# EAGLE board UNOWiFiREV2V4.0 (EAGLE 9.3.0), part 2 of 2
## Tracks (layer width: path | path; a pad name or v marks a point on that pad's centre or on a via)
2XTRANSLATOR1:N$1
  Top 0.254: C601.1 52.15,30.07 52.15,30.57 | U601.P$6 52.15,30.57 | R605.1 52.12,30.55 52.15,30.57
2XTRANSLATOR2:N$1
  Top 0.254: R405.1 60.25,10.75 59.88,11.12 58.05,11.12 C401.1
  Top 0.305: U401.P$6 55.65,10.3 55.9,10.55 58.02,10.55 C401.1
16XTRANSLATOR1:N$1
  Top 0.254: U504.2 43.42,17.43 42.95,16.95 R504.1
+3V3  (via drill 0.3, 0.35, 0.41)
  Top 0.254: C201.1 46.95,31.77 46.95,30.77 46.62,30.44 U201.8 | R301.2 61.35,29.35 v61.8,28.9 | v60.5,36.6 59.24,36.6 ON100.A | v34.75,22.5 30.73,22.5 30.02,23.2 v30.02,23.75 | C201.1 46.92,31.75 43.9,31.75 42.8,30.65 v42.8,30.62 | 48.38,31.4 v48.77,31.4 49.78,31.4 C202.1 49.85,31.2 49.88,31.2 R605.2 | 48.38,31.4 47.43,31.4 C201.1 | U201.5 48.3,31.32 48.38,31.4 | v48.92,18.38 49.23,18.07 U504.24 | v53.6,16.02 53.6,14.61 54.66,13.55 54.66,12.94 54.12,12.4 C402.1 53.45,11.25 52.5,10.3 U401.P$3 | U502.23 U502.24 50.12,26.48 v49.65,26.95 50.08,26.95 C505.1 | U504.24 51.15,18.07 51.39,17.83 51.39,16.99 v52.2,16.18 52.27,16.1 C506.1 | U504.23 U504.24 | 52.15,36.25 52.5,36.6 v53.9,36.6 54.4,36.1 C602.1 | 52.15,36.25 50.58,36.25 50.05,35.73 50.05,34.98 v50.23,34.8 | U601.P$3 52.15,36.25 | C301.1 R405.2
  Top 0.61: C301.1 63.5,10.75 | 63.5,10.75 C302.2 64.42,10.77 U301.10 64.41,12.5 63.51,12.5 v63.5,13.3 | U301.9 63.42,10.83 63.5,10.75
  Top 0.813: v28.1,13 28.5,13 30.66,10.84 34.1,7.4 v36.8,7.4 | R3.1 13.5,16.5 | 13.5,16.5 13,16.5 12.1,17.4 | 13.5,16.5 13.35,16.35 C105.1 14.58,14.62 v14.6,14.6
  Bottom 0.254: v53.9,36.6 v60.5,36.6 60.9,36.2 60.9,29.8 v61.8,28.9 | v34.75,22.5 35.16,22.5 36.15,23.45 36.45,23.75 36.45,24.59 36.8,24.95 36.8,25.64 37.64,26.47 38.33,26.47 40.11,28.24 41.8,29.93 42.1,29.93 v42.8,30.62 | v30.02,23.75 29.38,23.75 25.62,20 25.62,15.45 28.07,13 v28.1,13 | v53.6,16.02 53.45,16.18 v52.2,16.18 | v50.23,34.8 49.06,33.63 49.06,32.01 48.77,31.73 v48.77,31.4 48.77,27.82 v49.65,26.95 49.88,26.72 49.88,22.56 49.65,22.32 49.65,19.1 v48.92,18.38
  Bottom 0.813: v36.8,7.4 36.8,6.3 | v28.1,13 28.1,10.66 28.16,10.6 28.16,8.66 27.59,8.09 15.81,8.09 14.6,9.3 v14.6,14.6
  Bottom 1.016: POWER.4 35.56,5.06 36.8,6.3 37.3,6.8 61.1,6.8 62.88,8.57 63.5,9.2 v63.5,13.3
  other vias: 1.1,17.4 1.1,18.67 1.1,19.94 1.1,16.13 1.1,14.86 2.37,17.4 2.37,18.67 2.37,19.94 3.64,19.94 2.37,16.13 2.37,14.86 3.64,14.86 4.91,14.86 4.91,19.94 6.18,14.86 7.45,14.86 7.45,16.13 7.45,17.4 7.45,18.67 7.45,19.94 6.18,19.94
  pour Top: 0.4,20.7 9.3,20.7 9.3,18.6 12.6,18.6 12.6,16.3 9.3,16.3 9.3,14.1 0.4,14.1
  pour Bottom: 0.5,20.7 9.4,20.7 9.4,18.6 9.4,16.3 9.4,14.1 0.5,14.1
+5V  (via drill 0.3, 0.41)
  Top 0.305: Q101.D2 13.65,28.52 Q101.D2' | Q102.D2 11.58,28.27 Q102.D2'
  Top 0.61: Q102.D2' 12.7,28.39 | 12.7,28.39 13.77,28.39 Q101.D2' | v12.8,29.2 12.8,28.49 12.7,28.39 | v15.12,20.73 15.1,20.7 15.43,20.7 C104.1 17.08,21.33 C106.1
  Top 0.813: POWER.5 38.1,4.2 37.7,4.6 32.8,4.6 v27.2,10.2 | C104.1 15.93,21.2 R2.1 13.45,21.2 13.14,20.89 13.14,20.24 12.61,19.71 IC101.3
  Bottom 0.813: v12.8,29.2 12.4,28.8 12.4,23.45 v15.12,20.73 15.15,20.7 16.7,20.7 v27.2,10.2
GND  (via drill 0.3, 0.35)
  Top 0.254: U801.43 19.52,38.72 v19.3,38.5 19.3,36.79 U801.5 | U801.23 24.11,33.79 v23.8,34.1
  other vias: 47.58,30.75 21.5,36.3 23.8,38.5 19.3,34.1 18.27,33.08 61.5,24.8 10.4,22.1 21.95,40.65 40.75,37.9 24.9,32.15 23.05,29.82 24.82,24.85 22.5,44.88 24.88,42.5 21.12,43.08 37.98,46.75 40.42,46.75 47,46.75 54.67,46.75 51.67,46.75 64.95,45.05 67.7,22.2 64.5,24.5 60.15,33.17 55.5,13.65 60.5,14.93 19.12,28.3 26.8,29.82 43.85,36.5 14.88,31.88 25.9,37.9 17.6,42.15 18.2,43.95 54.05,27.1 44.15,41.3 45.4,25.73 39.4,32.2 45.25,33.12 58.6,39.12 59.92,5.33 57.42,5.33 54.88,5.28 62.35,23.25 19.12,13.88 20.12,13.88 21.73,14.38 17.52,18.57 49.3,25.07 49,17.43 49.77,29 48.98,19.77 45.55,29.2 52.75,20.27 53.02,21.75 28.18,35.45 51.17,20.5 19.15,25.77 22.8,26.1 25,19.3 46.02,16.45 36.92,29.68 24.6,15.8 26.77,15.45 16.57,46.67 48.02,32.75 42.1,27.75 44.25,30.12 33.17,10.9 31.48,11.8 40.8,13.53 36.2,16.77 45.5,19.6 39.77,18.05 37.83,13.53 45.3,17.5 51.4,13.65 43.02,11.18 45.5,14.35 53.3,33.95 47.33,13.05 58.52,13.62 55.48,19.25
  pour Bottom (rank 6): 0.64,53.34 67.69,53.34 68.58,52.45 68.58,0 0.89,0 0,0.89 0,46.35 0.64,46.35
  pour Top (rank 6): 0,53.34 68.58,53.34 68.58,0 0,0
  pour Top (rank 5, no thermals): 20.2,15.3 20.2,13.7 21.9,13.7 21.9,15.3
MEDBG1:N$1  (via drill 0.3)
  Top 0.406: D801.1 11.41,37.81 v11.4,37.55
  Top 0.61: R801.2 4.65,28.65 C801.1 3.82,29.48 USB801.SHIELD2 USB801.SHIELD1
  Bottom 0.406: v11.4,37.55 11.4,36.37 7.03,32 3.9,32 USB801.SHIELD2
MEDBG1:N$2
  Top 0.813: F801.2 9.17,36.2 USB801.VBUS
MEDBG1:N$3
  Top 0.61: C802.1 F801.1 L801.1
MEDBG1:N$4
  Top 0.254: U801.1 18.18,39.22 16.8,40.6 R802.1
MEDBG1:N$5
  Top 0.254: U801.6 14.27,36.28 C804.1
MEDBG1:N$6  (via drill 0.3)
  Top 0.254: U801.13 19.52,32.22 18.5,31.2 17.95,31.2 R803.1 17.82,30.98 v16.55,30.98 17,31.43 C805.1
  Bottom 0.254: v16.55,30.98 15.85,31.68 15.85,32.1 14.22,33.73 14.22,42.02 13.65,42.6 13.65,45.25 14.6,46.25 15.75,47.4 RST800.X
MEDBG1:N$7
  Top 0.254: U801.16 21.02,30.62 20.3,29.9 X801.1 19.8,27.2 19.05,26.45 C811.2
MEDBG1:N$8
  Top 0.254: U801.17 21.53,30.17 23.4,28.3 23.4,25.3 23.1,25 X801.3 21.9,23.12 C810.1
MEDBG1:N$9  (via drill 0.3)
  Top 0.254: R804.2 v25.5,29.3 | U801.20 23.03,31.07 v23.1,31.2
  Bottom 0.254: v25.5,29.3 25,29.3 v23.1,31.2
MEDBG1:N$10
  Top 0.254: R805.2 25.34,27.76 23.75,29.35 23.75,31.45 23.54,31.66 U801.21
MEDBG1:N$11
  Top 0.254: U801.27 26.34,35.77 LTX800.C
MEDBG1:N$12
  Top 0.254: U801.25 26.02,34.78 26.3,34.5 26.3,33.5 27.1,32.7 R806.1
MEDBG1:N$13
  Top 0.254: U801.26 26.14,35.29 LRX800.C
MEDBG1:N$14
  Top 0.254: R808.1 29.43,38.02 28.75,37.35 LTX800.A
MEDBG1:N$15
  Top 0.254: LRX800.A 30.2,34.3 30.45,34.55 R807.1
  Top 0.305: LRX800.A
MEDBG1:N$16
  Top 0.254: U801.33 26.72,38.77 R809.1 R810.2 29.4,38.85 TP801.X
MEDBG1:N$17  (via drill 0.3)
  Top 0.254: U801.11 16.91,33.79 v16.85,33.85 | v21.2,44.05 22.9,44.05 23.3,44.45 23.3,47.25 23.05,47.5 v21.75,47.5
  Bottom 0.254: v16.85,33.85 16.9,33.8 18.6,33.8 19.1,33.3 25.7,33.3 26.6,34.2 26.6,38.65 v21.2,44.05 | v21.75,47.5 MISO800.X
MEDBG1:N$18  (via drill 0.3)
  Top 0.254: U801.10 17.28,34.27 16.8,34.7 v16.35,34.7 | v16.8,45.2 16.8,43.2 16.6,43 16.05,43 v15.85,42.8
  Bottom 0.254: MOSI800.X 17.04,44.96 v16.8,45.2 | v16.35,34.7 16.1,34.95 16.1,41.5 16.5,41.9 16.5,42.85 16.35,43 16.05,43 v15.85,42.8
MEDBG1:N$19  (via drill 0.3)
  Top 0.254: U801.9 17.67,34.78 v17.15,35.2 | v16.8,48.25 18.25,48.25 v18.4,48.1 | v15.45,43.45 15.45,45.05 v14,46.5
  Bottom 0.254: v17.15,35.2 17.2,35.35 16.55,36 16.55,41.25 16.95,41.65 16.95,43.05 16.55,43.45 v15.45,43.45 | v18.4,48.1 18.4,47.61 SCK800.X | v16.8,48.25 16.75,48.25 16.65,48.35 15.47,48.35 14,46.88 v14,46.5
MEDBG1:USB2_N
  Top 0.254: U801.3 17.62,37.78 arc-45 16.92,38.07 R811.1
MEDBG1:USB2_PI
  Top 0.254: U801.4 16.39,37.27 arc-45 15.69,37.56 R812.1
MEDBG1:USB_N
  Top 0.254: 13.65,39.7 8.87,39.7 arc90 USB801.D- | D801.3 arc-90 13.65,40.51 13.65,39.7 | 13.65,39.7 14.87,39.7 arc-45 15.58,39.41 R811.2
MEDBG1:USB_P
  Top 0.254: USB801.D+ arc-90 6.58,39.31 6.58,38.7 arc90 7.13,38.15 9.23,38.15 arc90 9.78,38.7 9.78,39 arc-90 10.08,39.3 13.54,39.3 | D801.2 arc90 13.6,38.46 13.6,39.15 arc45 13.54,39.3 | 13.54,39.3 arc-45 14.25,39 R812.2
N$1  (via drill 0.3)
  Top 0.254: U301.20 60.42,19.55 v60.62,19.35 | v56.05,9.8 U401.P$5
  Bottom 0.254: v60.62,19.35 60.62,15.63 62.03,14.22 62.03,11.31 60.5,9.78 56.08,9.78 v56.05,9.8
N$2  (via drill 0.3)
  Top 0.254: v54.05,13.17 52.98,14.24 52.98,16.33 51.8,17.51 51.8,22.06 51.43,22.43 50.26,22.43 U502.18 | v54.77,12.2 55.14,12.2 U301.1
  Bottom 0.254: v54.77,12.2 54.62,12.35 54.05,12.92 v54.05,13.17
N$3
  Top 0.254: U301.22 58.42,21.43 57.25,22.6 52.04,22.6 51.44,23.2 U502.19
N$4  (via drill 0.3)
  Top 0.254: U301.36 56.38,19.85 v54.45,19.85 v54.45,19.84 | 50.83,14.82 v51.02,15.03 50.83,14.82 | U201.14 48.3,24.07 48.92,23.45 48.92,20.57 48.3,19.95 48.3,15.55 49.02,14.82 U504.19 50.83,14.82
  Bottom 0.254: v51.02,15.03 51.02,16.26 52.4,17.63 54.61,17.63 54.9,17.93 54.9,17.99 54.91,18 54.91,18.53 54.45,18.99 v54.45,19.84
N$5  (via drill 0.35)
  Top 0.254: U301.23 57.62,20.53 57.62,19.55 v57.7,19.48 | v48.55,14.38 48.75,14.18 U504.18
  Bottom 0.254: v48.55,14.38 48.55,14.93 54.07,20.45 56.73,20.45 v57.7,19.48
N$6
  Top 0.254: U201.1 49.08,28.06 49.35,28.06 49.43,27.99 49.43,27.61 48.72,26.9 48.72,24.36 49.31,23.77 50.06,23.77 U502.20
N$7  (via drill 0.3, 0.35)
  Top 0.254: U301.27 54.94,17.61 v54.3,18.25 | v50.05,9.8 U401.P$4
  Bottom 0.254: v54.3,18.25 52.44,18.25 49.16,14.96 49.16,14.12 48.38,13.34 48.38,11.15 49.73,9.8 v50.05,9.8
N$8  (via drill 0.35)
  Top 0.254: v54.38,16.5 54.3,16.57 54.34,16.61 U301.28 | v52.38,13.32 51.92,12.88 U504.16
  Bottom 0.254: v52.38,13.32 53.71,14.66 53.71,14.8 53.71,15.16 54.38,15.82 v54.38,16.5
N$9  (via drill 0.3)
  Top 0.254: v45.23,21.57 45.4,21.75 45.4,22.8 44.99,23.2 U502.6 | v42.11,14.03 42.11,12.83 41.55,12.28 IC1.2
  Bottom 0.254: v42.11,14.03 42.25,14.03 42.25,15.18 42.91,15.83 43.48,15.83 43.6,15.95 44.65,15.95 46.08,17.38 46.08,20.67 45.23,21.53 v45.23,21.57
N$10  (via drill 0.3)
  Top 0.254: v45.4,20.52 45.42,20.52 45.42,20.57 45.81,20.95 45.81,24.32 45.44,24.68 44.93,24.68 44.75,24.5 U502.4 | IC2.2 41.45,14.85 41.55,14.95 v41.52,14.95
  Bottom 0.254: v45.4,20.52 42.76,17.88 42.76,17.53 41.52,16.3 v41.52,14.95
N$12  (via drill 0.3)
  Top 0.254: R304.2 52.7,25.3 v52.4,25.6 | U601.P$5 51.65,32.02 v51.52,31.9
  Bottom 0.254: v52.4,25.6 51.95,25.6 51.25,26.3 51.25,31.62 v51.52,31.9
N$13  (via drill 0.3)
  Top 0.254: R303.2 52.65,24.3 v52.4,24.55 | U601.P$4 51.62,35.4 v50.83,35.4
  Bottom 0.254: v50.83,35.4 50.83,26.12 v52.4,24.55
N$14  (via drill 0.3, 0.35)
  Top 0.254: v32.17,25.55 32.33,25.4 33.9,25.4 34.83,26.33 U901.41 35.58,27 36.2,27 37.12,26.08 R901.1 38.23,26.04 v38.23,25.05 | R802.2 16.82,42.17 15.93,42.17 v15.78,42.02 | v21.93,28.7 21.88,28.7 v20.98,29.6 | R4.2 62.75,8.12 | 62.75,8.12 62.45,7.83 61.27,7.83 v60.6,8.5 | v45.45,27.41 v45.45,27.4 45.5,27.4 46.62,26.28 46.62,14.32 46.28,13.98 46.28,10.59 v46.35,10.53 | v63.23,6.88 63.23,7.65 62.75,8.12
  Bottom 0.254: v32.17,25.55 31.57,24.95 25.68,24.95 v21.93,28.7 | v20.98,29.6 20.4,29.6 18.3,31.7 18,31.7 15.65,34.05 15.65,41.85 v15.78,42.02 | v38.23,25.05 38.24,25.04 38.89,25.04 40.23,26.38 41.07,26.38 41.11,26.41 41.59,26.41 41.63,26.37 42.38,26.37 42.39,26.38 44.05,26.38 44.88,27.21 45.26,27.21 v45.45,27.41 | v60.6,8.5 46.3,8.5 45.35,9.45 45.35,9.94 45.76,10.35 46.17,10.35 v46.35,10.53 | JP1.1 49.05,6 62.85,6 63.25,6.4 63.25,6.9 v63.23,6.88
N$15
  Top 0.254: U201.4 50.76,29.66 51.3,29.12 51.3,26.5 51.3,24.7 51.02,24.43 50.22,24.43 U502.21
N$16
  Top 0.254: U201.12 47.3,27.74 47.45,27.59 47.45,23.78 48.11,23.11 48.11,20.91 47.45,20.25 47.45,13.85 49.73,11.57 U504.14
N$17  (via drill 0.3)
  Top 0.254: U801.29 25.66,36.79 v25.75,36.75 | v16.15,44.05 16.15,45.55 R903.2
  Bottom 0.254: v25.75,36.75 23.95,36.75 16.65,44.05 v16.15,44.05
N$18  (via drill 0.35)
  Top 0.254: v61.42,13.57 U301.7 | U502.17 50.22,21.82 v51.17,21.82
  Bottom 0.254: v61.42,13.57 60.68,14.32 58.12,14.32 57.77,14.66 57.77,15.22 57.79,15.24 57.79,15.27 58.13,15.61 58.16,15.61 58.34,15.79 58.34,19.83 57.13,21.04 51.96,21.04 v51.17,21.82
N$19
  Top 0.254: U901.9 27.43,25.97 26.35,27.05 R805.1
N$20
  Top 0.254: U901.8 27.8,26.4 27.3,26.9 27.3,27.48 R804.1
N$21  (via drill 0.3)
  Top 0.254: U901.26 32.75,19.25 32.42,19.57 31.73,19.57 v31.07,18.93 | USR.A 28.62,42.12 27.88,41.38 26.5,41.38 25.77,42.1 25.77,42.67 25.07,43.38 24.55,43.38 24.25,43.08 24.25,42.12 23.88,41.75 20.43,41.75 v19.95,42.23 | v26.9,18.02 24.5,18.02 23.35,19.18 v22.52,19.18 | v21.62,20.88 21.52,20.88 17.75,24.65 v17.75,24.75
  Bottom 0.254: v22.52,19.18 21.62,20.07 v21.62,20.88 | v17.75,24.75 17.57,24.93 17.57,31.55 15.15,33.98 15.15,42.35 14.7,42.8 14.7,45.05 15.45,45.8 18.8,45.8 19.15,45.45 19.15,43.02 v19.95,42.23 | v31.07,18.93 27.73,18.93 26.9,18.1 v26.9,18.02
N$22
  Top 0.254: USR.C R1.1
N$23  (via drill 0.3)
  Top 0.254: U201.13 47.8,27.84 47.88,27.77 47.88,23.93 48.52,23.28 48.52,20.74 47.88,20.1 47.88,14.03 49.67,12.22 U504.15 v51.48,12.22 | U301.29 54.59,15.61 54.3,15.32 v54.3,14.9
  Bottom 0.254: v54.3,14.9 54.3,14.38 52.15,12.22 v51.48,12.22
PA0  (via drill 0.3)
  Top 0.254: v36.3,30.15 36.3,29.82 33.86,27.39 U901.44
  Bottom 0.254: IOL.3 58.45,50.77 58.45,48.4 57.85,47.8 53.75,47.8 50.95,45 50.05,45 36.3,31.25 v36.3,30.15
PA1  (via drill 0.3)
  Top 0.254: v35.1,31.15 34.7,30.75 34.7,28.9 33.54,27.74 U901.45
  Bottom 0.254: IOL.8 45.72,41.87 35.1,31.25 v35.1,31.15
PA2  (via drill 0.3)
  Top 0.254: IOH.9 20.33,49.79 U701.5 21.53,46.47 v22.27,45.73 | v34.1,31.38 34.1,29.1 33.13,28.14 U901.46 | v32.88,35.73 35.58,35.73 v36.7,34.6 37.15,34.15 v40.05,34.15 | v42.7,35.9 44.45,34.15 52.42,34.15 53.15,34.88 U601.P$1
  Bottom 0.254: v34.1,31.38 34.1,32 v36.7,34.6 | v42.7,35.9 41.8,35.9 v40.05,34.15 | v22.27,45.73 22.88,45.73 32.67,35.92 v32.88,35.73
PA3  (via drill 0.3)
  Top 0.254: v39.62,33.42 37.02,33.42 v36.73,33.73 35.4,35.05 32.65,35.05 32.2,35.5 32.2,36.1 32.65,36.55 v32.65,36.85 | U701.6 19.83,47.4 v19.68,47.55 19.68,49.92 IOH.10 | v42.7,34.8 43.77,33.73 52.48,33.73 53.15,33.05 U601.P$8 | v35,32 33.83,32 33.5,31.68 33.5,29.17 U901.47
  Bottom 0.254: v35,32 v36.73,33.73 | v42.7,34.8 41.33,33.42 v39.62,33.42 | v32.65,36.85 22.95,46.55 20.25,46.55 19.68,47.12 v19.68,47.55
PA4  (via drill 0.3)
  Top 0.254: v32.92,30.32 33.02,30.32 33.02,29.4 U901.48 | v35.09,33.81 35.5,33.4 35.58,33.4 38.33,30.64 38.33,29.99 39.52,28.81 | 39.52,28.81 | 39.52,28.81 39.76,28.57 | 39.76,28.57 | v42.14,26.95 41.37,26.95 39.76,28.57 | v42.14,26.95 v42.15,26.95 v42.14,26.95 | v45.44,28.34 45.72,28.06 45.73,28.06 47.04,26.75 47.04,23.61 47.71,22.95 47.71,21.09 47.04,20.43 47.04,13.9 v46.87,13.72 | U504.6 44.26,14.8 v43.52,14.8
  Bottom 0.254: v35.09,33.81 v35.1,33.8 35.1,33.6 32.91,31.41 v32.91,30.33 v32.92,30.32 | v42.14,26.95 43.9,26.95 44.98,28.03 44.97,28.03 45.27,28.34 v45.44,28.34 | v46.87,13.72 44.83,13.72 43.75,14.8 v43.52,14.8
PA5  (via drill 0.3)
  Top 0.254: v29.6,29.75 29.6,29.47 U901.1 | v41.35,25.82 37.51,29.67 37.51,30.32 35.62,32.21 35.24,32.58 33.78,32.58 32.32,31.12 v32.25,31.12 | U502.5 44.95,23.85 v45.2,24.1
  Bottom 0.254: v41.35,25.82 40.77,25.24 40.77,24.71 41.25,24.23 45.08,24.23 v45.2,24.1 | v32.25,31.12 30.5,31.12 29.6,30.23 v29.6,29.75
PA6  (via drill 0.35)
  Top 0.254: U401.P$1 51.25,11.3 51.09,11.46 v51.09,11.49 | U901.2 30.52,27.84 v30.52,27.07 | v23.15,21.93 23.15,23.85 24.24,24.94 24.24,25.09 24.58,25.43 24.73,25.43 v25.57,26.27 | v26.23,13.85 28.77,13.85 29.04,13.58 30.22,13.58 30.73,13.07 31.3,13.07 32.42,11.96 33.07,11.96 34.58,10.45 34.58,10.15 v34.73,10 | v47.45,11.1 48.67,11.1 v49,11.43
  Bottom 0.254: v30.52,27.07 30.13,26.68 29.11,26.68 28.7,26.27 v25.57,26.27 | v23.15,21.93 23.15,20.53 22.95,20.33 22.95,19.57 23.11,19.42 23.11,15.72 24.81,14.01 24.84,14.01 24.96,13.89 25.44,13.89 25.45,13.9 26.18,13.9 v26.23,13.85 | v34.73,10 44.83,10 45.97,11.13 47.42,11.13 v47.45,11.1 | v51.09,11.49 49.07,11.49 v49,11.43
PA7  (via drill 0.35)
  Top 0.254: U901.3 29.02,28.63 29.02,28.65 28.6,29.07 28.6,29.79 v28.85,30.04 | v43.11,40.12 43.11,39.17 45.77,36.51 49.61,36.51 51.67,38.58 54.2,38.58 55.48,37.3 55.48,35.48 56.17,34.77 56.17,33.5 | 56.17,33.5 56.17,32.33 R302.1 | Q301.2 58.62,33.28 58.4,33.5 56.17,33.5
  Bottom 0.254: v43.11,40.12 39.98,40.12 31.39,31.53 30.33,31.53 v28.85,30.05 v28.85,30.04
PB0  (via drill 0.3)
  Top 0.254: U901.4 28.18,28.77 v28.18,30.48
  Bottom 0.254: 39.05,39.83 39.05,50.73 IOH.2 | 39.05,39.83 | 39.05,39.83 32.51,33.28 31.64,33.28 30.68,32.32 30.53,32.32 29.3,31.09 28.77,31.09 28.18,30.49 v28.18,30.48
PB1  (via drill 0.3)
  Top 0.254: v28.18,31.32 27.5,30.65 27.5,28.75 U901.5
  Bottom 0.254: IOH.3 36.58,37.93 32.34,33.69 31.47,33.69 30.54,32.76 30.39,32.76 29.13,31.5 28.35,31.5 v28.18,31.32
PB2  (via drill 0.3)
  Top 0.254: v29.35,26.1 29.35,26.19 U901.6
  Bottom 0.254: IOL.6 50.8,46.38 35.92,31.45 35.7,31.23 35.7,29.9 32.85,27.05 32.2,27.05 31,25.85 29.6,25.85 v29.35,26.1
PB3  (via drill 0.3)
  Top 0.254: U901.7 27.71,27.12 27.71,27.92 25.74,29.88 v25.27,30.35 | v24.27,27.98 23.81,27.51 23.81,25.11 23.07,24.37 23.07,24.34 22.52,23.79 22.52,21.68 23.07,21.13 23.07,20.06 24.5,18.62 v26.21,18.62 | v26.23,16.77 27.97,16.77 29.15,15.59 31.04,15.59 32.88,13.75 32.87,13.74 32.87,12.98 v32.9,12.95 | v43.23,12.43 43.42,12.22 U504.10 | IC2.1 40.33,14.2 40.23,14.1 | 40.23,14.1 40.12,14 40.12,13.1 v39.9,12.88 | R5.1 40.61,16.56 40.1,16.05 40.1,14.3 40.23,14.18 40.23,14.1
  Bottom 0.254: v25.27,30.35 25.74,29.88 26.08,29.54 26.08,29.06 25.74,28.72 25.02,28.72 v24.27,27.98 | v26.21,18.62 26.21,16.79 v26.23,16.77 | v32.9,12.95 33,12.85 39.88,12.85 v39.9,12.88 40.35,12.43 v43.23,12.43
PC0  (via drill 0.3)
  Top 0.254: v45.92,15.2 45.9,15.18 45.5,15.18 45.2,15.47 U504.5 | v23.77,21.35 23.8,21.35 23.8,22.52 25.74,24.47 25.74,25.27 26.38,25.91 26.72,25.91 27,25.62 U901.10 | v25.2,14.47 28.72,14.47 29.21,13.99 30.41,13.99 30.89,13.51 31.45,13.51 32.59,12.37 33.23,12.37 33.33,12.27 v33.77,12.27
  Bottom 0.254: SPI1.4 65.12,27.94 64.06,26.89 62.19,26.89 59.51,24.21 58.21,24.21 56.51,22.51 51,22.51 50.46,21.97 50.46,17.44 48.4,15.38 47.92,15.38 | v25.2,14.47 25.1,14.47 23.53,16.04 23.53,20.34 23.77,20.57 v23.77,21.35 | 47.92,15.38 47.92,13.59 47.92,12.76 47.01,11.84 40.11,11.84 39.51,12.44 33.95,12.44 v33.77,12.27 | v45.92,15.2 46.1,15.38 47.42,15.38 47.92,15.38
PC1  (via drill 0.3)
  Top 0.254: v24.96,21.9 v24.95,21.9 24.95,22.48 27.02,24.56 27.02,24.89 26.73,25.18 U901.11 | v31.23,14.57 31.27,14.61 31.27,14.62 30.72,15.18 28.97,15.18 27.97,16.18 25.07,16.18 v24.59,16.65 | IC1.4 39.08,13 39.68,13.6 39.68,14.87 IC2.4 39.05,16 v39.02,16.02 | v37.14,16.97 36.02,18.08 36.02,18.7 v36.01,18.68
  Bottom 0.254: SPI1.1 61.31,32.8 61.31,36.62 60.44,37.48 52.96,37.48 51.55,36.08 50.65,36.08 48.65,34.08 48.65,32.17 48.17,31.7 48.17,25.66 44.98,22.46 43.46,22.46 41.45,20.45 38.72,20.45 36.97,18.69 36.05,18.69 35.92,18.69 | v31.23,14.57 31.23,16.59 33.33,18.69 35.92,18.69 | v24.59,16.65 24.48,16.65 23.94,17.18 23.94,20.17 24.96,21.18 v24.96,21.9 | v39.02,16.02 38.08,16.02 v37.13,16.97 v37.14,16.97 | 35.92,18.69 35.99,18.69 v36.01,18.68
PC2  (via drill 0.3)
  Top 0.254: v33.45,13.5 33.45,13.78 31.23,15.99 29.32,15.99 27.89,17.43 v24.57,17.43 | v45.2,12.93 45.15,12.88 U504.9 | U901.12 26.38,24.51 24.35,22.48 24.35,20.12 v24.55,19.93
  Bottom 0.254: SPI1.3 62.66,27.94 59.34,24.61 58.04,24.61 56.36,22.94 50.85,22.94 50.06,22.14 50.06,17.61 48.25,15.8 45.65,15.8 45.27,15.43 43.07,15.43 42.73,15.09 42.73,14.19 | 24.39,19.07 24.39,19.77 v24.55,19.93 | 24.39,19.07 24.39,17.6 v24.57,17.43 | v33.45,13.5 33.67,13.28 36.72,13.28 37.79,14.35 39.24,14.35 40.85,14.35 41.73,13.47 41.77,13.43 42.35,13.43 42.73,13.81 42.73,14.19 | v45.2,12.93 v45.19,12.92 45.03,12.92 43.76,14.19 42.73,14.19 | 24.39,19.07
PC4  (via drill 0.3)
  Top 0.254: v30.85,21.45 30.85,21.8 29.5,23.15 28.75,23.15 28,22.4 28,22.2 27.5,21.7 U901.16 | v60.95,44.65 IOL.2
  Bottom 0.254: v30.85,21.45 31.6,21.45 33.5,23.35 35.42,23.35 35.42,23.37 36.04,23.99 36.04,24.79 36.4,25.14 36.4,25.81 37.47,26.88 38.13,26.88 47.57,36.27 47.95,36.27 56.33,44.65 v60.95,44.65
PC5  (via drill 0.3)
  Top 0.254: v29.9,21.9 29.3,22.5 28.77,22.5 28.45,22.15 28.45,21.9 27.84,21.34 U901.17
  Bottom 0.254: IOL.1 63.45,50.75 63.45,48.2 60.9,45.65 56.76,45.65 47.78,36.68 47.56,36.68 | v29.9,21.9 30.05,22.05 31.15,22.05 32.9,23.8 34.5,23.8 34.52,23.82 35.29,23.82 35.63,24.16 35.63,24.98 35.99,25.34 35.99,25.98 37.3,27.28 37.94,27.28 47.34,36.68 47.56,36.68 | 47.56,36.68
PC6  (via drill 0.3)
  Top 0.254: IOL.5 53.34,46.24 v49.35,42.25 | v29.05,21.9 U901.18
  Bottom 0.254: v49.35,42.25 49,42.25 47.62,40.88 47.65,40.85 47.65,38.85 37.3,28.5 36.8,28.5 34.77,26.48 34.77,25.97 34,25.2 33.7,25.2 31,22.5 29.65,22.5 v29.05,21.9
PC7  (via drill 0.3)
  Top 0.254: v27.67,18.04 27.71,18.04 27.77,18.1 27.77,19.91 U901.19 | v29.45,14.57 30.4,14.57 30.99,13.98 31.82,13.98 31.82,13.97 31.81,13.99 v31.8,13.99 | v43.33,20.72 42.48,20.72 41.58,21.62 41.58,23.03 43.7,25.15 U502.3
  Bottom 0.254: v29.45,14.57 29.45,16.26 v27.67,18.04 | v29.45,14.57 | v31.8,13.99 31.8,14.31 31.81,14.33 31.81,16.6 33.3,18.08 36.93,18.08 38.89,20.04 41.62,20.04 41.64,20.06 42.41,20.06 43.23,20.88 43.35,20.88 43.35,20.75 v43.33,20.72
PD0
  Top 0.254: U901.20 28.86,20.26 28.25,19.65 28.25,17.65 29.5,16.4 31.4,16.4 34.36,13.44 34.36,13.3 34.36,11.29 38.55,7.1 48.5,7.1 50.8,4.8 AD.1
PD1
  Top 0.254: U901.21 29.21,19.91 28.7,19.4 28.7,17.9 29.75,16.85 31.65,16.85 34.77,13.73 34.77,13.3 34.77,11.46 38.72,7.51 48.79,7.51 53.3,3 53.3,2.58 AD.2
PD2
  Top 0.254: U901.22 29.15,19.15 29.15,18.15 30,17.3 31.9,17.3 35.17,14.03 35.17,11.63 38.89,7.91 51.04,7.91 55.9,3.05 55.9,2.56 AD.3
PD3
  Top 0.254: U901.23 29.6,18.9 29.6,18.4 30.25,17.75 32.15,17.75 35.66,14.24 35.66,11.71 39.05,8.32 53.13,8.32 58.5,2.95 58.5,2.62 AD.4
PD4
  Top 0.254: AD.5 61,2.58 61,3 55.27,8.73 39.22,8.73 36.1,11.85 36.1,14.5 32.43,18.17 30.97,18.17 U901.24
PD5
  Top 0.254: U901.25 36.56,14.74 36.56,11.96 39.39,9.13 57.22,9.13 63.5,2.85 AD.6
PD7  (via drill 0.3)
  Top 0.152: U901.27 33.25,19.5
  Top 0.254: C1.1 C2.1 23.88,43.75 IOH.8 | 33.25,19.5 33.42,19.32 33.42,18.45 36.97,14.91 36.97,13.4 36.97,12.43 v37.98,11.43
  Bottom 0.152: 23.75,51 IOH.8
  Bottom 0.254: v37.98,11.43 34.38,11.43 34.02,11.07 34.02,1.43 33.34,0.75 18.5,0.75 14.18,5.08 10.7,5.08 8.88,6.9 8.88,12.2 10.75,14.07 10.75,19.25 8.25,21.75 8.25,31.88 13,36.62 13,51.65 14.11,52.75 22,52.75 23.75,51
PE0  (via drill 0.3)
  Top 0.254: IOH.4 34.04,47.6 40.34,41.3 v40.6,41.3 | U901.30 34.16,20.64 33.8,21 33.5,21 v33.1,21.4 | v43.1,41.3 42.5,40.7 42.5,39.1 45.5,36.1 48.27,36.1 48.42,35.95 v48.42,35.9 | v41,21.05 41,23.12 43.15,25.27 43.15,30.12 44.17,31.15 v45.98,31.15
  Bottom 0.254: v43.1,41.3 v40.6,41.3 | v45.98,31.15 45.98,33.75 48.12,35.9 v48.42,35.9 | v33.1,21.4 33.1,21.12 34.95,19.27 35.88,19.27 36.98,19.27 37.44,19.74 37.51,19.81 38.75,21.05 v41,21.05
PE1  (via drill 0.3)
  Top 0.254: U901.31 34.55,20.9 34.84,20.62 34.84,20.11 34.86,20.09 v34.95,20.18 | IOH.5 31.48,50.78 31.48,45.5 41.34,35.64 41.34,35.63 41.34,30.33 42.12,29.55 v42.12,29.12
  Bottom 0.254: v34.95,20.18 34.95,21.32 36.88,23.25 36.88,24.43 37.21,24.76 37.21,25.47 37.8,26.06 38.51,26.06 41.6,29.15 42.1,29.15 v42.12,29.12
PE2  (via drill 0.3)
  Top 0.254: U901.32 35.58,20.67 35.58,20.1 v35.8,19.88 | IOH.6 28.96,47.24 40.92,35.27 40.92,30.45 40.92,30.18 41.54,29.56 41.54,28.4 v41.7,28.4
  Bottom 0.254: v35.8,19.88 35.8,20.15 35.59,20.36 35.59,21.27 37.27,22.95 37.27,23.07 37.28,23.08 37.28,24.23 37.62,24.57 37.62,25.3 37.97,25.66 38.71,25.66 41.45,28.4 v41.7,28.4
PE3  (via drill 0.3)
  Top 0.254: IOH.1 41.66,50.59 41.75,50.5 41.75,30.5 42.73,29.52 42.73,25.45 40.35,23.07 v40.35,21.65 | v36.17,20.6 36.17,20.78 U901.33
  Bottom 0.254: v36.17,20.6 36.23,20.55 37.67,20.55 38.8,21.68 40.33,21.68 v40.35,21.65
PF2
  Top 0.254: U901.36 36.85,22.23 38.72,22.23 41.59,19.35 41.59,17.5 42.12,16.97 42.12,14.86 42.7,14.27 42.7,13.53 | 42.7,13.53 42.7,12.85 41.48,11.62 IC1.1 40.62,11.6 R11.1 | U504.8 43.4,13.53 42.8,13.53 42.7,13.53
PF3  (via drill 0.3)
  Top 0.254: v42.67,22.5 44.26,22.5 U502.7 | v37.88,23.6 37.63,23.6 U901.37
  Bottom 0.254: v42.67,22.5 38.98,22.5 v37.88,23.6
PF4  (via drill 0.3)
  Top 0.254: U901.38 v35.05,24.4 | v48.25,40.35 IOL.7
  Bottom 0.254: v48.25,40.35 v48.26,40.34 48.26,37.73 47.64,37.12 47.2,37.12 37.77,27.69 37.13,27.69 35.59,26.14 35.59,25.5 35.23,25.15 35.23,25.03 35.05,24.85 v35.05,24.4
PF5  (via drill 0.3)
  Top 0.254: U901.39 35.61,25.56 35.17,25.12 35.05,25 34.8,25 34.27,24.48 v34.27,24.4 | v47.4,37.7 55.85,46.1 55.85,50.77 IOL.4
  Bottom 0.254: v47.4,37.7 47.15,37.7 37.55,28.09 36.96,28.09 35.18,26.31 35.18,25.68 34.27,24.77 v34.27,24.4
PWR1:N17690335  (via drill 0.3)
  Top 0.305: R127.2 13.45,27.16 Q101.S2 13.4,27.11 v13.4,26.7 | Q101.S1 15.24,29.44 v15.4,29.6
  Bottom 0.305: v15.4,29.6 15.4,30 14.6,30.8 13.8,30.8 13.65,30.65 13.65,26.95 v13.4,26.7
PWR1:N17690346  (via drill 0.3)
  Top 0.305: Q101.G1 v14.3,30.1 | v14.3,25.1 14.3,25.85 R127.1 14.3,25.95 Q101.G2 | Q105.6 13.4,22 v14.3,22.9
  Bottom 0.305: v14.3,30.1 v14.3,25.1 v14.3,22.9
PWR1:N17690381
  Top 0.305: Q105.2 12.1,24.5 12.3,24.7 | 12.3,24.7 13.8,24.7 14.1,24.4 15.02,24.4 R125.1 | R126.2 12.37,24.77 12.3,24.7
PWR1:N17690821  (via drill 0.3)
  Top 0.305: R128.2 9.57,26.64 Q102.S1 10.2,27.27 v10.2,26.5 | Q102.S2 11.58,30.32 v11.1,30.8
  Bottom 0.305: v10.2,26.5 10.2,29.9 v11.1,30.8
PWR1:N17690840
  Top 0.254: 10.79,25.74 10.89,25.74 10.93,25.7 | Q102.G2 10.93,30.05 10.45,30.52 9.6,30.52 8.22,29.15 8.22,25.9 8.38,25.75 R128.1
  Top 0.305: Q102.G1 10.93,25.7 | R128.1 10.79,25.74 | 10.93,25.7 10.93,24.22 Q105.3 | R126.1 11.13,25.9 10.93,25.7
PWR1:N17690878
  Top 0.305: C114.1 R124.2 R123.1 10.25,23.15 10.6,22.8 12,22.8 12.1,22.7 Q105.5
PWR1:N$1
  Top 0.254: 11.89,8.1 11.82,8.1 11.82,7.68 J201.+2 | J201.+3 J201.+1
  Top 1.422: D101.A 18.11,2.79 12.8,8.1 11.89,8.1 J201.+1
PWR1:N$3  (via drill 0.3, 0.41)
  Top 0.254: IC105.7 15.9,15.55 15.9,17.9 17.2,19.2 18.05,19.2 R102.2
  Top 0.305: Q102.D1 10.28,28.52 Q102.D1'
  Top 0.61: Q102.D1' 9.19,28.39 v9,28.2 | R123.2 9.8,21.45 9.8,21.3 9.78,21.3 v9.76,21.29
  Bottom 0.61: v9,28.2 9,22.05 v9.76,21.29 12.61,21.29 17.9,16 17.9,15.1
  other vias: 17.1,13.4 18.1,13.4 17.1,12.4 17.1,11.4 17.1,10.4
  pour Top (rank 5, no thermals): 16.55,15.5 15.95,15.5 15.95,9.9 16,9.85 20.4,9.85 20.4,13.2 18.4,13.2 18.4,15.5 16.6,15.5
  pour Bottom (rank 5, no thermals): 16.55,15.5 15.95,15.5 15.95,9.9 16,9.85 20.4,9.85 20.4,13.2 18.4,13.2 18.4,15.5 16.6,15.5
PWR1:N$4
  Top 0.254: R101.1 ON100.C
PWR1:N$35
  Top 0.254: IC105.1 20.35,19.2 20.35,19.7 20.3,19.75 | R102.1 19.65,19.75 20.3,19.75 | R129.2 20.3,19.75
PWR1:N$36
  Top 0.254: IC105.17 21.85,16.95 22.3,17.4 22.8,17.4 R130.2
PWR1:N$37
  Top 0.254: IC105.18 21.25,18.27 R131.2
TRG_RST  (via drill 0.3)
  Top 0.254: C903.1 v39.53,24.46 39.18,24.8 R902.1 39.18,24.88 38.55,24.24 37.98,24.24 35.97,26.26 35.63,26.26 35.34,25.97 U901.40 35.17,25.97 34.19,24.99 32.45,24.99 32.42,24.97 31.93,24.97 31.15,25.75 31.15,27.84 31.49,28.18 31.51,28.18 31.77,28.45 31.77,29.18 32.02,29.43 v32.02,30.12 | R904.1 15.45,47.16 R903.1 15.5,47.8 16.6,48.9 18.55,48.9 19.09,48.36 v19.09,48.49 | v29.49,33.48 29.48,33.47 R806.2 30.04,32.71 30.24,32.51 30.24,30.14 v30.29,30.09 | SPI1.5 v60.55,28.48 | v57.27,32.7 57.3,32.68 Q301.3 | v43.33,21.49 42.9,21.92 42.43,21.92 42.09,22.26 42.09,22.74 42.97,23.62 v43.25,23.62 | v56.27,38.1 56.27,35.6 57.27,34.6 v57.25,34.6
  Bottom 0.254: v19.09,48.49 21.86,48.49 33.51,36.84 33.51,35.53 33.12,35.14 32.86,34.88 30.76,34.88 29.48,33.6 29.49,33.58 v29.49,33.48 | v60.55,28.48 59.23,29.79 59.23,30.54 58.89,30.88 58.14,30.88 57.27,31.75 v57.27,32.7 57.25,32.73 v57.25,34.6 | v30.29,30.09 31.99,30.09 v32.02,30.12 | POWER.3 32.3,3.26 32.3,13.66 32.38,13.74 32.38,16.6 33.46,17.68 37.1,17.68 39.06,19.64 43.06,19.64 43.91,20.48 43.91,20.97 43.9,20.98 43.9,21.38 43.8,21.48 43.38,21.48 43.36,21.49 v43.33,21.49 | v39.53,24.46 v39.52,24.45 40.35,23.62 v43.25,23.62 43.38,23.5 45.43,23.5 46.99,25.07 46.99,30.99 47.12,31.13 47.12,32.27 47.44,32.59 47.44,33.44 50.49,36.49 51.34,36.49 51.69,36.83 51.69,36.84 52.95,38.1 v56.27,38.1
UC1:N$2
  Top 0.254: PB901.3 10,47.15 | 10,47.15 PB901.4 | R904.2 10,47.16 10,47.15
UC1:N$3
  Top 0.254: C905.1 37.11,18.62 Y901.1
  Top 0.305: U901.34 37.11,20.55 Y901.1
UC1:N$4
  Top 0.254: C904.1 39.18,20.87 Y901.2
  Top 0.305: U901.35 37.5,20.87 37.95,20.87 Y901.2
UPDI_REMOTE  (via drill 0.3)
  Top 0.254: U401.P$8 55.3,11.3 v55.48,11.12 | v61.85,9.55 R4.1
  Bottom 0.254: v55.48,11.12 55.47,11.12 55.47,9.56 55.81,9.22 61.54,9.22 61.85,9.53 v61.85,9.55
VDD  (via drill 0.3)
  Top 0.254: C809.2 19.05,40.3 | 19.05,40.3 19.05,39.64 U801.44 | U801.24 25.63,34.27 25.8,34.1 25.8,33.2 26.8,32.2 | 26.8,32.2 C807.1 | R808.2 R807.2 31.35,35.05 v32.1,34.3 | v27.06,23.48 27.06,22.73 U901.14 25.67,21.34 C907.2 25.9,21.58 v25.9,21.99 v25.89,22 | v32.6,20.79 32.62,20.79 U901.28 34.36,19.06 C906.2 | 26.8,32.2 27.3,32.2 v27.5,32 | 24.9,39.63 U801.34 24.02,41.03 23.75,41.3 20.8,41.3 | 24.9,39.63 26.68,39.63 R809.2 v26.8,40.65 | C808.2 24.9,39.63 | 17.95,30.3 R803.2 | v18.5,40.3 19.05,40.3 | U801.14 20.03,31.93 18.8,30.7 v18.8,30.3 | U701.8 18.56,46.2 C701.2 17.55,43.25 19.05,41.75 C809.2 | 20.8,41.3 20,41.3 | 20,41.3 C809.2 | U801.42 20,39.63 20,41.3 | v20.75,40.8 20.75,41.25 20.8,41.3 | v17.2,38.8 17.2,38.5 17.45,38.25 18.14,38.25 U801.2 | v41.35,24.95 40.65,24.95 39.88,25.72 R902.2 R901.2 38.44,26.9 38,26.9 37.8,26.7 37.4,26.7 37.02,27.08 C902.2 C901.1 35.85,27.98 U901.42 33.87,26 v33.12,26 32.55,26 31.73,26.82 v31.73,27.6 | v45.12,26.62 45.12,26.38 | v42.17,17.77 42.1,17.77 42.17,17.85 R504.2 | v40.55,17.48 40.52,17.45 40.12,17.45 39.73,17.05 R5.2 39.63,16.61 38.61,16.61 38.42,16.42 38.42,15.19 39.05,14.55 IC2.5 38.44,14.19 38.44,12.26 IC1.5 39.73,10.97 R11.2 39.73,9.82 39.95,9.6 45.85,9.6 45.85,9.62 v45.95,9.72 47.14,9.72 C403.1 | R504.2 42.95,18.07 U504.1 45.05,18.07 46.22,19.24 46.22,25.81 45.65,26.38 45.12,26.38 | C503.1 R504.2 | 45.12,26.38 44.38,26.38 U502.1 44.27,26.48 C504.1 v43.73,27.62 | U601.P$7 52.65,31.95 52.88,31.73 53.98,31.73 v54.42,32.17 C603.1 55.15,32.75 55.77,33.37 55.77,34.61 55.05,35.33 55.05,36.35 54.23,37.17 54.15,37.17 54.14,37.18 51.21,37.18 v51.1,37.07
  Top 0.254: U401.P$7 53.58,10.8 52.62,9.85 52.74,9.73 v52.74,9.72
  Top 0.305: C806.1 R803.2 | 17.95,30.3 v18.8,30.3 | v30.43,33.48 30.9,33 30.9,30.95 30.9,30.35 30.9,30.3 30.9,29.35 v30.75,29.2 | SPI1.2 66.15,30.5 66.15,31.5 63.7,33.95 v59.35,33.95
  Top 0.406: v26.35,19.75 26.3,19.8 26.3,20.6 25.71,21.19 C907.2
  Top 0.61: R2.2 16.43,19.6 17.83,21 v20,21
  Top 0.813: R3.2 R2.2
  Bottom 0.254: v17.2,38.8 17.2,39 v18.5,40.3 | v27.5,32 27.5,39.95 v26.8,40.65 | VDD800.X 20.83,44.68 20.4,44.25 20.4,42.65 20.55,42.5 20.55,41 v20.75,40.8 | 26,22 | v43.73,27.62 43.6,27.62 43.6,28.62 45.54,30.57 46.22,30.57 46.56,30.91 46.56,33.76 48.08,35.27 48.68,35.27 50.48,37.07 v51.1,37.07 | v42.17,17.77 41.88,17.48 v40.55,17.48 | v52.74,9.72 52.23,9.2 46.47,9.2 v45.95,9.72 | v41.35,24.95 42.34,25.94 44.44,25.94 v45.12,26.62
  Bottom 0.305: v27.5,32 26.7,31.2 24.05,31.2 23.3,31.95 22.8,31.95 21.73,30.88 21.73,29.4 20.56,28.24 | v59.35,33.95 58.08,35.23 56.55,35.23 54.42,33.1 v54.42,32.17
  Bottom 0.406: v18.8,30.3 18.8,30 20.55,28.25 20.56,28.24 20.56,26.89 24.24,23.21 25.43,23.21 | v32.1,34.3 30.88,34.3 30.43,33.85 v30.43,33.48 28.95,32 v27.5,32 27.5,28.75 28.75,27.5
  Bottom 0.61: 25.43,23.21 25.43,22.73 21.8,22.73 20.07,21 v20,21
  Bottom 0.813: POWER.2 30.3,2.54 30.3,2.8 30.36,14.28 30.38,16.98 31.04,17.6 | v26.35,19.75 28.18,21.57
  pour Bottom: 24.24,23.35 31.29,30.4 37.87,23.82 30.82,16.77
VIN
  Top 1.27: POWER.8 45.7,2.56 45.7,3.8 43.4,6.1 33.7,6.1 28.26,11.54 C101.+
  pour Top (rank 5, no thermals): 20.8,16.6 23.8,16.6 23.8,13.3 26.5,13.3 26.5,9.7 23.7,9.8 23.7,4.4 25.1,4.4 25.1,1.1 22.4,1.1 22.4,9.7 22.4,16.3 20.8,16.3
VUSB  (via drill 0.3)
  Top 0.254: L801.2 15.25,35.35 15.75,35.85 17.4,35.85 17.5,35.75 18.16,35.75 U801.7
  Top 0.305: Q101.D1 14.95,27.95 15.4,28.4
  Top 0.605: C803.1 15.85,32.7 15.35,32.7 v14.4,32.7
  Top 0.61: R125.2 15.8,26.08 15.8,28.3 15.7,28.4 | Q101.D1' 15.4,28.4 15.7,28.4 | 15.7,28.4 16.2,28.9 16.2,30.2 15.8,30.6 15.05,30.6 14.65,31 13.95,31 13.6,31.35 13.6,32.45 13.85,32.7 v14.4,32.7 | L801.2 15.25,32.8 15.35,32.7 | D801.4 11.6,41.3 12.1,41.8 v13.6,41.8
  Bottom 0.605: v14.4,32.7 13.6,33.5 v13.6,41.8
WIFI/BLE1:N$1
  Top 0.254: U301.19 61.42,19.78 61.6,19.6 64.8,19.6 65.1,19.9 65.1,23.1 | 65.1,23.1 65.1,28.7 64.5,29.3 62.5,29.3 61.6,30.2 60.95,30.2 R301.1 60.65,30.25 60,30.9 59.39,30.9 Q301.6 | C303.1 65.1,23.1
WIFI/BLE1:N$2  (via drill 0.3)
  Top 0.254: R303.1 57.5,24.3 v59,22.8 | U301.35 56.91,18.3 57.73,18.3 58.3,18.88 v58.95,19.52
  Bottom 0.254: v59,22.8 59,19.57 v58.95,19.52
WIFI/BLE1:N$3  (via drill 0.3)
  Top 0.254: R304.1 57.6,25.3 59.9,23 v59.9,22.2 | U301.31 57.32,13.86 58.38,14.91 v58.38,15.03
  Bottom 0.254: v59.9,22.2 59.9,18.65 59.9,16.55 v58.38,15.03
WIFI/BLE1:N$4
  Top 0.305: U301.16 64.4,20.76 64.4,21.8 63.9,22.3 62.9,22.3 62.51,22.3 62.28,22.53 61.5,22.53 61.5,23.6 60.4,24.7 60.4,27.5 59.96,27.94 DL301.2
WIFI/BLE1:N$5
  Top 0.305: DL301.1 59.2,26.62 59.2,25.1 61.01,23.29 61.01,22.34 61.27,22.07 62.09,22.07 62.36,21.8 63,21.8 63.42,21.38 U301.17
WIFI/BLE1:N$6
  Top 0.305: 58,25.6 58,28.6 58.39,28.99 DL301.3 | U301.18 62.4,20.76 62.4,21.1 62.08,21.42 62.08,21.44 61.9,21.61 61.09,21.61 60.55,22.15 60.55,23.05 58,25.6 | 58,25.6
WIFI/BLE1:N$7
  Top 0.305: DL301.5 54.29,27.94 R305.2
WIFI/BLE1:N$8
  Top 0.305: DL301.6 54.84,26.89 R306.2
WIFI/BLE1:N$9
  Top 0.305: DL301.4 54.96,28.99 R307.2
WIFI/BLE1:N$10  (via drill 0.3)
  Top 0.254: U301.24 56.42,21.82 v56.5,21.9 | v67.6,23.1 67.6,31.5 v66.7,32.4 | R309.2 v63.1,32.55
  Bottom 0.254: v67.6,23.1 67.1,22.6 61,22.6 59.8,23.8 58.38,23.8 56.5,21.93 v56.5,21.9 | v66.7,32.4 63.25,32.4 v63.1,32.55
WIFI/BLE1:N$11  (via drill 0.3)
  Top 0.254: R310.1 52.8,23.3 51.82,24.28 51.82,26.52 v52.4,27.1 | v58.65,30.3 58.65,30.85 Q301.5 58.65,30.91 58.65,31.5 58.75,31.6 60.75,31.6 R308.1
  Top 0.305: R309.1 R308.1
  Bottom 0.254: v58.65,30.3 58.65,29.25 55.65,26.25 53.9,26.25 53.05,27.1 v52.4,27.1
WIFI/BLE1:N$12
  Top 0.254: R310.2 57.63,23.3 59.4,21.57 59.4,20.76 U301.21

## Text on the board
tPlace: 13 | 12 | 11 | 10 | 9 | 8 | 7 | 6 | 5 | 4 | 3 | 2 | 1 | 0
tNames: AREF | GND | # | # | # | # | # | # | DIGITAL | TX1 | RX1 | 1 | ANALOG IN | IOREF | RESET | 3V3 | 5V | GND | VIN | A0 | A1 | A2 | A3 | A4 | A5
214bmp: D:/SmartProjects/Snc/a4_bn_logo2.bmp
